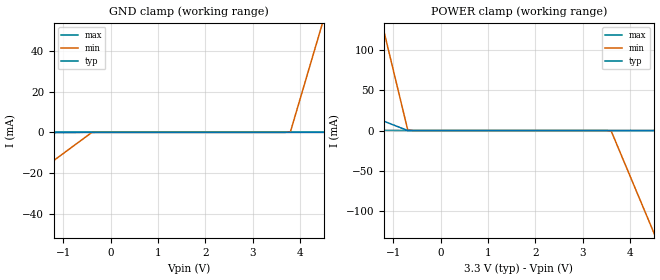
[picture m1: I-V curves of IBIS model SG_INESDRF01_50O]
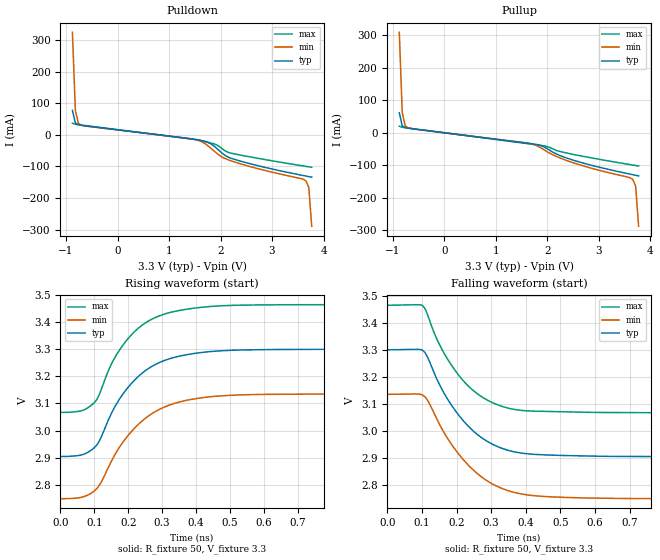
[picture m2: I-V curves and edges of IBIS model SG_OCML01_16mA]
|   This file is an IBIS representation of the   |
|   Integrated Device Technology, Inc.   |
|   ICS858S011   |
|   LOW SKEW, 1-TO-2 DIFFERENTIAL-TO-CML FANOUT BUFFER   |
[IBIS Ver]   4.1
[File name]   858s011i.ibs
[File Rev]   3.0
[Date]   16 Jul 2010
[Source]   Originated at Integrated Device Technology, Inc.
[Notes]
IN and nIN each have an internal 50ohm termination to VT. The Series model code can be
used to simulate that.  Aside from the code below, the 50ohm terminations were
not modeled, so the user can use external components to model this correclty.
The Diff Pin property above is used for that pin pair in order to allow the
similator to verify that the input swing is sufficient.
It is recommended that the user manually add the two 50ohm resistors external
to the device and provide the biasing voltage.  This will correctly model
the behavior of the input while giving the user control over the bias voltage
at the center node of the input pair.
[Disclaimer]
IDT hereby grants the user of this IBIS model a non-exclusive,
nontransferable license to use this IBIS model under the following terms.
Before using this IBIS model, the user should read this license.
If the user does not accept these terms,  the IBIS model should be
returned to IDT within 30 days.
   The user is granted this license only to use the IBIS model and
is not granted rights to sell, load, rent, lease or license the IBIS
model in whole or in part, or in modified form to anyone other than
user. User may modify the IBIS model to suit its specific
applications but rights to derivative works and such modifications
shall belong to IDT.
   This IBIS model is provided on an "AS IS" basis and IDT makes
absolutely no warranty with respect to the information contained
herein. IDT DISCLAIMS AND CUSTOMER WAIVES ALL WARRANTIES, EXPRESS
OR IMPLIED, INCLUDING WARRANTIES OF MERCHANTABILITY OR FITNESS FOR
A PARTICULAR PURPOSE. The entire risk as to quality and performance
is with the Customer. ACCORDINGLY, IN NO EVENT SHALL THE COMPANY BE
LIABLE FOR ANY DAMAGES, WHETHER IN CONTRACT OR TORT,INCLUDING ANY
LOST PROFITS OR OTHER INCIDENTAL, CONSEQUENTIAL, EXEMPLARY, OR
PUNITIVE DAMAGES ARISING OUT OF THE USE OR APPLICATION OF THE IBIS
model provided in this package. Further, IDT reserves the right to
make changes without notice to any product herein to improve
reliability, function, or design. IDT does not convey any license
under patent rights or any other intellectual property rights,
including those of third parties.
   IDT is not obligated to provide maintenance or support
for the licensed IBIS model.
[Copyright]   Copyright 2010 by Integrated Device Technology, Inc.
[Component]   ICS858S011KI
[Manufacturer] Integrated Device Technology, Inc.
[Package]
|LD QFN 16
|lead + wire   typ   min   max
R_pkg   72.4655m   58.886m   86.045m
L_pkg   1.47175nH   1.11650nH   1.77850nH
C_pkg   0.07747pF   0.07444pF   0.08050pF
[Pin] signal_name  model_name   R_pin   L_pin   C_pin
1   IN   SG_INESDRF01_50O   86.045m   1.77850nH   0.08050pF
2   VT   NC   58.886m   1.11650nH   0.07444pF
3   VREF_AC   POWER   58.886m   1.11650nH   0.07444pF
4   nIN   SG_INESDRF01_50O   86.045m   1.77850nH   0.08050pF
5   VCC   POWER   86.045m   1.77850nH   0.08050pF
6   VEE   GND   58.886m   1.11650nH   0.07444pF
7   VEE   GND   58.886m   1.11650nH   0.07444pF
8   VCC   POWER   86.045m   1.77850nH   0.08050pF
9   Q1   SG_OCML01_16mA   86.045m   1.77850nH   0.08050pF
10   nQ1   SG_OCML01_16mA   58.886m   1.11650nH   0.07444pF
11   nQ0   SG_OCML01_16mA   58.886m   1.11650nH   0.07444pF
12   Q0   SG_OCML01_16mA   86.045m   1.77850nH   0.08050pF
13   VCC   POWER   86.045m   1.77850nH   0.08050pF
14   VEE   GND   58.886m   1.11650nH   0.07444pF
15   VEE   GND   58.886m   1.11650nH   0.07444pF
16   VCC   POWER   86.045m   1.77850nH   0.08050pF
[Diff Pin]  inv_pin  vdiff tdelay_typ tdelay_min  tdelay_max
1   4   0.30   NA   NA   NA
9   10   NA   0   0   0
12   11   NA   0   0   0
| Models and submodels in the file (2): SG_INESDRF01_50O (Input), SG_OCML01_16mA (Output_ECL)
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|IN and nIN each have an internal 50ohm termination to VT. The code below can be
|used to simulate that.  Aside from the code below, the 50ohm terminations were
|not modeled, so the user can use external components to model this correclty.
|The Diff Pin property above is used for that pin pair in order to allow the
|similator to verify that the input swing is sufficient.
|It is recommended that the user manually add the two 50ohm resistors external
|to the device and provide the biasing voltage.  This will correctly model
|the behavior of the input while giving the user control over the bias voltage
|at the center node of the input pair.
|[Series Pin Mapping] Pin_2   model_name   function_table_group
| ODT between IN and nIN =100 ohm
|1   4   ODT_100
| Similators might not support ODT=50ohm on IN to nVT amd nIN to VT
|1   2   ODT_50
|4   2   ODT_50
|[Model]   ODT_50
|Model_type  Series
|Polarity   Non-Inverting
|   typ   min   max
|C_comp   0pF   0pF   0pF
|   typ   min   max
|[Voltage Range]  3.3V   3.135V   3.465V
|   typ   min   max
|[R Series]   50ohm   45ohm   55ohm
|[Model]   ODT_100
|Model_type  Series
|Polarity   Non-Inverting
|   typ   min   max
|C_comp   0pF   0pF   0pF
|   typ   min   max
|[Voltage Range]   3.3V   3.135V   3.465V
|   typ   min   max
|[R Series]   100ohm   90ohm   110ohm
[Model]   SG_INESDRF01_50O
Model_type   Input
Polarity   Non-Inverting
Vinl = 0.8V
Vinh = 2.0V
|   typ   min   max
C_comp   2pF   1.5pF   2.5pF
|   typ   min   max
[Voltage range]   3.3V   3.135V   3.465V
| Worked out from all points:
|   POWER clamp passes 1 mA (typ) near -0.74 V on its own axis
[GND_clamp]
|Voltage   I (typ)   I (min)   I (max)
-3.3V     -547.9uA   -49.76mA   -354.4nA
-400mV    -393.2nA   -69.82uA   -94.11pA
3.8V      19.97nA    321uA      15.87pA
4.4V      5.769uA    47.58mA    23.32pA
4.5V      6.727uA    55.46mA    24.56pA
6.6V      26.85uA    220.9mA    50.61pA
[Power_clamp]
|Voltage   I (typ)   I (min)   I (max)
-3.3V     59.92mA    637.5mA    1.293mA
-1.3V     13.86mA    147.9mA    298.7uA
-1.2V     11.56mA    123.4mA    249uA
-700mV    47.95uA    997.7uA    345.1nA
-500mV    19.97nA    1.53uA     33.25pA
3.6V      -8.028nA   -573.7uA   -7.74pA
4.5V      -3.474uA   -127.3mA   -13.35pA
4.6V      -3.859uA   -141.4mA   -13.97pA
6.6V      -11.56uA   -422.9mA   -26.43pA
[Model]   SG_OCML01_16mA
Model_type   Output_ECL
Polarity   Non-Inverting
|   typ   min   max
C_comp   2pF   1.5pF   2.5pF
Vmeas = 3.1V
Rref = 50
Cref = 0
Vref = 3.3V
|   typ   min   max
[Voltage range]   3.3V   3.135V   3.465V
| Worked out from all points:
|   rising waveform, R_fixture 50, V_fixture 3.3: 20-80 % time 127ps typ, 137ps min, 118ps max; typ from 2.9 V to 3.3 V
|   falling waveform, R_fixture 50, V_fixture 3.3: 20-80 % time 130ps typ, 138ps min, 122ps max; typ from 3.3 V to 2.9 V
[Pulldown]
|Voltage   I (typ)   I (min)   I (max)
|Note, modeling breaks down at 250mA and above.  This is well beyond the functional   |
|operating range of the device.  Should this scenario occur, catastrophic failure and   |
|possible damage to the device and/or board is of higher concern than the I-V curve   |
|behavior.  The IBIS checker will flag currents in excess of 10A with warnings.  Lines   |
|with currents in excess of 0.35 A have been commented out.  The points still remain|
|available to the user if the user desires to use them.   |
|-2.84000e+00   1.70534e+08   1.39103e+08   2.23175e+08
|-2.38000e+00   1.18995e+08   9.61989e+07   1.57268e+08
|-1.92000e+00   6.74566e+07   5.32943e+07   9.13610e+07
|-1.46000e+00   1.59179e+07   1.03898e+07   2.54538e+07
|-1.00000e+00   5.67126e+00   1.54360e+01   1.09104e+00
|-9.90000e-01   3.86357e+00   1.14693e+01   6.77512e-01
|-9.32644e-01   4.45116e-01   1.90740e+00   7.24056e-02
-875.3mV  77.42mA    324.5mA    36.45mA
-817.9mV  36.95mA    76.71mA    33.26mA
-760.6mV  31.58mA    37.15mA    31.96mA
-645.9mV  28.78mA    27.98mA    29.58mA
1.534V    -15.31mA   -16.45mA   -15.77mA
1.82V     -29.58mA   -43.81mA   -26.58mA
1.993V    -52.86mA   -66.68mA   -39.2mA
2.165V    -71.97mA   -80.18mA   -56.67mA
3.599V    -128.9mA   -140.5mA   -98.56mA
3.656V    -130.8mA   -145.3mA   -100.1mA
3.713V    -132.6mA   -166.2mA   -101.5mA
3.771V    -134.4mA   -289.9mA   -103mA
| 3.82793e+00   -1.36293e-01   -1.07260e+00   -1.04499e-01
| 3.88529e+00   -1.38563e-01   -5.70934e+00   -1.05968e-01
| 3.94264e+00   -1.44780e-01   -2.81651e+01   -1.07432e-01
| 4.00000e+00   -1.87903e-01   -1.62120e+02   -1.08891e-01
| 4.01000e+00   -2.10252e-01   -2.22330e+02   -1.09145e-01
| 4.52800e+00   -2.07102e+06   -8.21251e+06   -1.16810e+04
| 5.04600e+00   -5.79948e+07   -6.31817e+07   -5.20111e+07
| 5.56400e+00   -1.24026e+08   -1.18151e+08   -1.36451e+08
| 6.08200e+00   -1.90057e+08   -1.73120e+08   -2.20891e+08
| 6.60000e+00   -2.56089e+08   -2.28089e+08   -3.05332e+08
[Pullup]
|Voltage   I (typ)   I (min)   I (max)
|Note, modeling breaks down at 250mA and above.  This is well beyond the functional   |
|operating range of the device.  Should this scenario occur, catastrophic failure and   |
|possible damage to the device and/or board is of higher concern than the I-V curve   |
|behavior.  The IBIS checker will flag currents in excess of 10A with warnings.  Lines   |
|with currents in excess of 0.35 A have been commented out.  The points still remain|
|available to the user if the user desires to use them.   |
|-2.84000e+00   1.70534e+08   1.39103e+08   2.23175e+08
|-2.38000e+00   1.18995e+08   9.61989e+07   1.57268e+08
|-1.92000e+00   6.74566e+07   5.32943e+07   9.13610e+07
|-1.46000e+00   1.59179e+07   1.03898e+07   2.54538e+07
|-1.00000e+00   5.65554e+00   1.54205e+01   1.07483e+00
|-9.90000e-01   3.84772e+00   1.14540e+01   6.61290e-01
|-9.32644e-01   4.29265e-01   1.89215e+00   5.61865e-02
-875.3mV  61.57mA    309.2mA    20.24mA
-817.9mV  21.1mA     61.46mA    17.05mA
-760.6mV  15.74mA    21.89mA    15.75mA
-645.9mV  12.94mA    12.73mA    13.37mA
1.648V    -33mA      -32.44mA   -34.11mA
1.878V    -39.75mA   -46.89mA   -38.87mA
2.165V    -64.62mA   -72.03mA   -53.89mA
2.451V    -81.74mA   -89.61mA   -64.83mA
3.599V    -127mA     -138.2mA   -97.77mA
3.656V    -128.9mA   -143.1mA   -99.28mA
3.713V    -130.8mA   -164.1mA   -100.8mA
3.771V    -132.7mA   -287.8mA   -102.3mA
| 3.82793e+00   -1.34583e-01   -1.07058e+00   -1.03760e-01
| 3.88529e+00   -1.36891e-01   -5.70742e+00   -1.05241e-01
| 3.94264e+00   -1.43146e-01   -2.81635e+01   -1.06716e-01
| 4.00000e+00   -1.86306e-01   -1.62119e+02   -1.08185e-01
| 4.01000e+00   -2.08661e-01   -2.22329e+02   -1.08440e-01
| 4.52800e+00   -2.07102e+06   -8.21251e+06   -1.16810e+04
| 5.04600e+00   -5.79948e+07   -6.31817e+07   -5.20111e+07
| 5.56400e+00   -1.24026e+08   -1.18151e+08   -1.36451e+08
| 6.08200e+00   -1.90057e+08   -1.73120e+08   -2.20891e+08
| 6.60000e+00   -2.56089e+08   -2.28089e+08   -3.05332e+08
[Ramp]
|   typ   min   max
dV/dt_r   0.237/0.127n   0.231/0.137n   0.238/0.118n
dV/dt_f   0.238/0.129n   0.232/0.138n   0.24/0.122n
R_load =   50.0000
[Rising Waveform]
R_fixture = 50
V_fixture = 3.3
V_fixture_min = 3.135
V_fixture_max = 3.465
C_fixture = 0.0p
| Time   typ   min   max
0s        2.904V     2.748V     3.067V
63.06ps   2.91V      2.754V     3.073V
100.1ps   2.937V     2.777V     3.103V
117.1ps   2.967V     2.802V     3.14V
153.2ps   3.07V      2.893V     3.253V
192.2ps   3.148V     2.97V      3.328V
245.2ps   3.216V     3.04V      3.393V
307.3ps   3.259V     3.087V     3.43V
494.5ps   3.296V     3.13V      3.462V
1ns       3.3V       3.135V     3.465V
[Falling Waveform]
R_fixture = 50
V_fixture = 3.3
V_fixture_min = 3.135
V_fixture_max = 3.465
C_fixture = 0.0p
| Time   typ   min   max
0s        3.3V       3.135V     3.465V
103.1ps   3.297V     3.131V     3.462V
119.1ps   3.265V     3.107V     3.42V
154.2ps   3.162V     3.015V     3.31V
209.2ps   3.053V     2.909V     3.201V
265.3ps   2.981V     2.836V     3.132V
335.3ps   2.933V     2.784V     3.089V
399.4ps   2.915V     2.763V     3.074V
490.5ps   2.909V     2.754V     3.071V
1ns       2.904V     2.748V     3.067V
